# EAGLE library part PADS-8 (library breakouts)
PIN HEADER
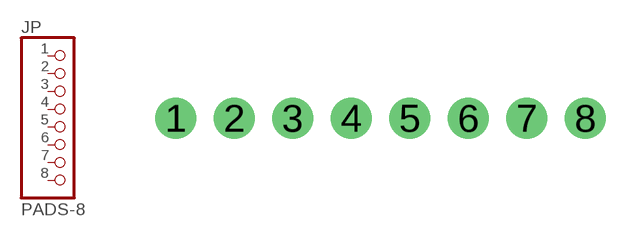
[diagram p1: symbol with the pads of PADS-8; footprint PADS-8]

Designator prefix JP

## PADS-8CLEANBIG  [PADS-8]
1  1  pas
2  2  pas
3  3  pas
4  4  pas
5  5  pas
6  6  pas
7  7  pas
8  8  pas

## Footprint PADS-8 (pad centres in mm)
drill 1.016 pad 1.778: 1 -8.89,0; 2 -6.35,0; 3 -3.81,0; 4 -1.27,0; 5 1.27,0; 6 3.81,0; 7 6.35,0; 8 8.89,0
